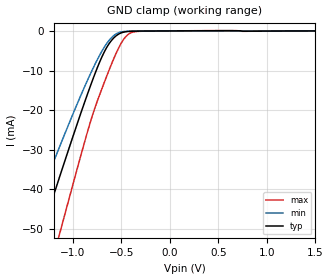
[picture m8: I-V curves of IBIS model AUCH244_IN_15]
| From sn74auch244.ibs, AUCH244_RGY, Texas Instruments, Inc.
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[Model]   AUCH244_IN_15
Model_type  Input
Vinl=0.49
Vinh=1.04
| variable   typ   min   max
C_comp   2.52pF   2.01pF   2.83pF
[Temperature Range]   40   100   -40
| Ambient temperature   25   85   -40
[Voltage range]   1.5   1.4   1.6
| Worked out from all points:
|   GND clamp passes 1 mA (typ) near -0.54 V on its own axis
[GND Clamp]
| AUCH244_IN_15
|   Voltage   I(typ)   I(min)   I(max)
-3.6V     -227.9mA   -191.3mA   -273.5mA
-1.475V   -62.59mA   -50.36mA   -82.08mA
-1.34V    -52.23mA   -41.81mA   -69.76mA
-1.3V     -49.18mA   -39.3mA    -66.11mA
-1.14V    -37.07mA   -29.41mA   -51.5mA
-1.09V    -33.33mA   -26.37mA   -46.95mA
-825mV    -14.26mA   -11.13mA   -23.41mA
-690mV    -5.975mA   -4.646mA   -13.87mA
-570mV    -1.564mA   -999.4uA   -6.496mA
-435mV    -146.6uA   -80.85uA   -978.7uA
-280mV    -39.88uA   -25.15uA   -76.46uA
1.5V      176.5pA    533.5nA    75.27pA
